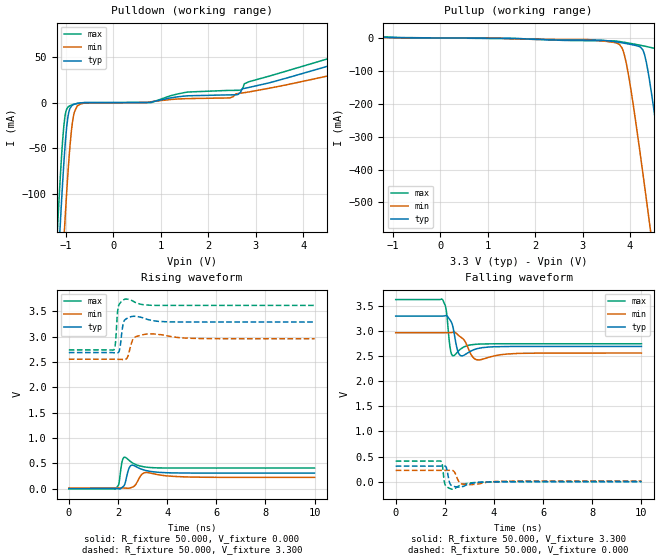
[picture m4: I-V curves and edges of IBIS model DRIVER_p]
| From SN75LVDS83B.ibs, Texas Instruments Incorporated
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[Model]   DRIVER_p
Model_type   Output
Polarity   Non-Inverting
Enable   Active-Low
Vmeas = 1.65
Vref = 1.65
Cref = 15pF
Rref = 50
|   typ   min   max
C_comp   0.250e-12   NA   NA
|C_comp (ON state)   1.000e-200   NA   NA
|C_comp (OFF state)   1.000e-200   NA   NA
[Voltage Range]   3.3   2.97   3.63
[Temperature Range]   25   125   -40
[Pullup Reference]   3.3   2.97   3.63
[Pulldown Reference]   -0   -0   -0
[Power Clamp Reference]   3.3   2.97   3.63
[GND Clamp Reference]   -0   -0   -0
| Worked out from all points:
|   slope of the pulldown table from 0 to 0.495 V, typ, clamps not added: 8.25 kohm
|   slope of the pullup table from 0 to 0.495 V, typ, clamps not added: 1.57 kohm
|   falling waveform, R_fixture 50.000, V_fixture 3.300: 20-80 % time 164ps typ, 333ps min, 111ps max; typ from 3.29 V to 2.69 V
|   rising waveform, R_fixture 50.000, V_fixture 0.000: 20-80 % time 108ps typ, 158ps min, 73ps max; typ from 0.004 V to 0.31 V
|   rising waveform, R_fixture 50.000, V_fixture 3.300: 20-80 % time 90.4ps typ, 134ps min, 70.2ps max; typ from 2.69 V to 3.29 V
|   falling waveform, R_fixture 50.000, V_fixture 0.000: 20-80 % time 71.4ps typ, 110ps min, 56.6ps max; typ from 0.31 V to 0.004 V
[Pulldown]
|   Voltage   I(typ)   I(min)   I(max)
-3.3V     -2.605A    -2.686A    -2.562A
-1.201V   -212.5mA   -304.6mA   -159.4mA
-1.171V   -182.3mA   -274mA     -129.6mA
-1.132V   -143.3mA   -233.9mA   -91.76mA
-1.043V   -64.15mA   -148mA     -24.09mA
-1.023V   -49.45mA   -130.1mA   -15.57mA
-963.6mV  -17.21mA   -80.38mA   -5.378mA
-864.6mV  -2.962mA   -21.74mA   -2.342mA
-825mV    -1.939mA   -10.66mA   -1.696mA
-696.3mV  -551.7uA   -1.658mA   -424.6uA
2.62V     8.74mA     9.723mA    13.31mA
6.59V     75.72mA    51.76mA    81.84mA
[Pullup]
|   Voltage   I(typ)   I(min)   I(max)
-3.3V     18.74mA    12.69mA    24.32mA
3.729V    -12.22mA   -15.8mA    -9.677mA
3.838V    -14.8mA    -32.56mA   -11.98mA
3.937V    -17.34mA   -88.2mA    -14.42mA
4.283V    -40.71mA   -424.9mA   -23.95mA
4.422V    -139.1mA   -575.2mA   -28.25mA
4.6V      -319.4mA   -772.6mA   -34.82mA
4.699V    -426.3mA   -883.5mA   -55.29mA
4.798V    -535.5mA   -995.1mA   -132.3mA
4.887V    -634.9mA   -1.096A    -221.4mA
5.224V    -1.016A    -1.48A     -591.2mA
6.59V     -2.595A    -3.057A    -2.167A
[Ramp]
R_load = 50
|   typ   min   max
dV/dt_r   0.185944/1.07719e-010  0.134605/1.58458e-010  0.245766/7.3295e-011
dV/dt_f   0.36179/1.62451e-010  0.248232/3.34879e-010  0.515447/1.11384e-010
[Falling Waveform]
R_fixture = 50.000
V_fixture = 3.300
V_fixture_min = 2.970
V_fixture_max = 3.630
C_fixture = 0.000
|  time   V(typ)   V(min)   V(max)
0s        3.292V     2.961V     3.62V
1.898ns   3.292V     2.961V     3.624V
2.045ns   3.303V     2.961V     3.442V
2.21ns    3.215V     2.962V     2.677V
2.314ns   3.106V     2.969V     2.505V
2.505ns   2.63V      2.932V     2.573V
2.649ns   2.503V     2.873V     2.64V
3.375ns   2.651V     2.42V      2.735V
4.938ns   2.688V     2.549V     2.742V
10ns      2.689V     2.558V     2.742V
[Rising Waveform]
R_fixture = 50.000
V_fixture = 0.000
V_fixture_min = 0.000
V_fixture_max = 0.000
C_fixture = 0.000
|  time   V(typ)   V(min)   V(max)
0s        4.21mV     15.85mV    614.4pV
1.898ns   4.542mV    16.07mV    -4.341mV
2.032ns   -397.4uV   16.09mV    88.05mV
2.15ns    19.98mV    16.1mV     495mV
2.275ns   88.44mV    14.14mV    624.5mV
2.417ns   360.8mV    10.82mV    576.5mV
2.549ns   465.7mV    26.29mV    525.1mV
3.126ns   362.6mV    322.6mV    429.1mV
4.738ns   311.7mV    234.8mV    409.7mV
10ns      309.9mV    225.2mV    409.6mV
[Rising Waveform]
R_fixture = 50.000
V_fixture = 3.300
V_fixture_min = 2.970
V_fixture_max = 3.630
C_fixture = 0.000
|  time   V(typ)   V(min)   V(max)
0s        2.689V     2.558V     2.742V
1.831ns   2.686V     2.558V     2.742V
1.902ns   2.684V     2.558V     2.899V
2.005ns   2.687V     2.556V     3.574V
2.066ns   2.745V     2.555V     3.653V
2.206ns   3.247V     2.552V     3.726V
2.274ns   3.333V     2.552V     3.741V
2.63ns    3.405V     2.968V     3.699V
3.197ns   3.344V     3.056V     3.627V
10ns      3.292V     2.961V     3.62V
[Falling Waveform]
R_fixture = 50.000
V_fixture = 0.000
V_fixture_min = 0.000
V_fixture_max = 0.000
C_fixture = 0.000
|  time   V(typ)   V(min)   V(max)
0s        309.9mV    225.2mV    410.5mV
1.844ns   311.5mV    226.5mV    407.2mV
1.898ns   312.2mV    226.6mV    334.9mV
2.005ns   311.2mV    226.7mV    -51.63mV
2.083ns   244.8mV    226.7mV    -101mV
2.181ns   966.4uV    226.8mV    -128.8mV
2.275ns   -73.34mV   226.9mV    -146.3mV
2.63ns    -104.9mV   -31.65mV   -67.98mV
2.911ns   -57.53mV   -54.96mV   -33.18mV
10ns      4.21mV     15.85mV    -8.284uV
